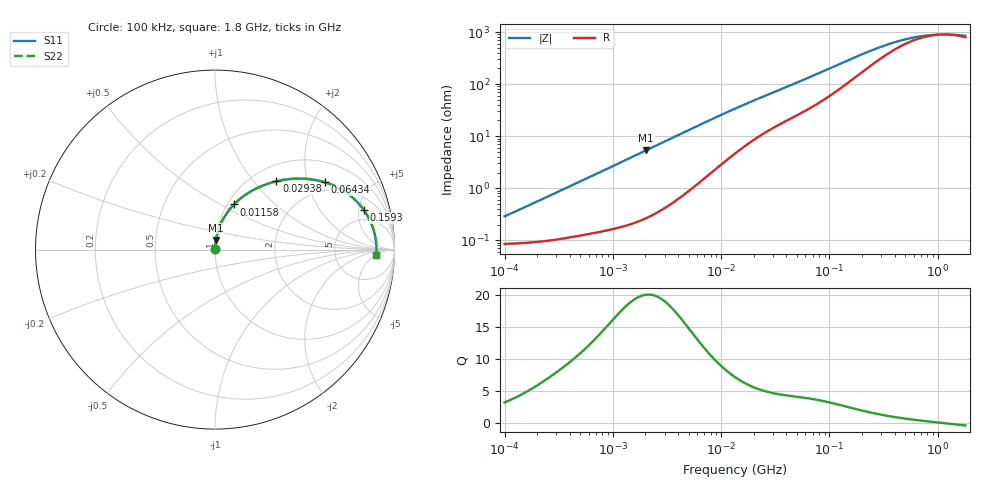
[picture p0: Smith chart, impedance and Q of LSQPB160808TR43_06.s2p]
! LSQPB160808TR43_06  S-PARAMETER MODEL  ( General Type )
! Model Generated by TAIYO YUDEN Corporation (http://www.ty-top.com)
! Version 1.0
! TAIYO YUDEN Control No. 110726NG25SE-FKC
! Copyright(c) 2011 TAIYO YUDEN CO.,LTD. All Rights Reserved.
! Product Description (link to TY-COMPAS)
! https://ds.yuden.co.jp/TYCOMPAS/or/detail?pn=LSQPB160808TR43M06&u=M
! Products Name : Inductors
! Characteristics :
!  Inductance : 0.43 uH , SRF(min) : 740 MHz , DC Resistance(max) : 0.1066 Ohm
!  Rated Current : Saturation :1400 mA , Temp Rise : 1100 mA (40 degC)
!  Case Size : 1.6 x 0.8 / 0.063 x 0.031 [mm/inch] , Thickness : 0.8 / 0.031 [mm/inch]
!  (Conditions: Temperature = 25 degC , DC Bias Current/Voltage = 0A / 0V)
! External Node Assignments :
!  1  o---GGG---o  2
! GND o---------o GND
! Frequency Range : 0.1MHz  -  1800MHz  [ 402 STEP ]
# MHz S RI R 50
! Freq[MHz].  S11 Real  S11 Imag  S21 Real  S21 Imag  S12 Real  S12 Imag  S22 Real  S22 Imag
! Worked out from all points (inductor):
!   401 points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, 100 kHz to 1.8 GHz, reference 50 ohm
!   read as one part in series: L = 438 nH near 105 kHz
!   highest Q = 20.1 at 2.035 MHz (marker M1), where L = 419 nH
!   self-resonance near 1.146 GHz
!   S11 on the Smith chart (normalised r, x): 100 kHz: 1.00, +0.01; 11.58 MHz: 1.07, +0.58; 29.38 MHz: 1.28, +1.32; 64.34 MHz: 1.67, +2.59; 159.3 MHz: 3.37, +5.64; 1.8 GHz: 17, -6
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0.1  0.000857 0.00275  0.9991 -0.00275  0.9991 -0.00275  0.000857 0.00275
0.144402  0.000896 0.00397  0.9991 -0.00397  0.9991 -0.00397  0.000896 0.00397
0.516129  0.00144 0.0139  0.9986 -0.0139  0.9986 -0.0139  0.00144 0.0139
2.034681  0.0055 0.0531  0.9945 -0.0531  0.9945 -0.0531  0.0055 0.0531
2.66389  0.00837 0.0692  0.9916 -0.0692  0.9916 -0.0692  0.00837 0.0692
6.278453  0.0375 0.1548  0.9625 -0.1548  0.9625 -0.1548  0.0375 0.1548
8.632747  0.0655 0.2024  0.9345 -0.2024  0.9345 -0.2024  0.0655 0.2024
11.58263  0.106 0.2517  0.894 -0.2517  0.894 -0.2517  0.106 0.2517
13.41641  0.1327 0.2769  0.8673 -0.2769  0.8673 -0.2769  0.1327 0.2769
19.37354  0.2183 0.3346  0.7817 -0.3346  0.7817 -0.3346  0.2183 0.3346
29.38042  0.3426 0.3806  0.6574 -0.3806  0.6574 -0.3806  0.3426 0.3806
44.5561  0.4853 0.3956  0.5147 -0.3956  0.5147 -0.3956  0.4853 0.3956
64.33982  0.6134 0.3747  0.3866 -0.3747  0.3866 -0.3747  0.6134 0.3747
69.24595  0.6375 0.3665  0.3625 -0.3665  0.3625 -0.3665  0.6375 0.3665
105.0131  0.754 0.3005  0.246 -0.3005  0.246 -0.3005  0.754 0.3005
159.2548  0.8284 0.2216  0.1716 -0.2216  0.1716 -0.2216  0.8284 0.2216
229.9669  0.8648 0.1588  0.1352 -0.1588  0.1352 -0.1588  0.8648 0.1588
357.3983  0.8863 0.0992  0.1137 -0.0992  0.1137 -0.0992  0.8863 0.0992
542.0029  0.8953 0.057  0.1047 -0.057  0.1047 -0.057  0.8953 0.057
802.0705  0.8988 0.0254  0.1012 -0.0254  0.1012 -0.0254  0.8988 0.0254
1186.925  0.8998 -0.00247  0.1002 0.00247  0.1002 0.00247  0.8998 -0.00247
1800  0.8987 -0.0326  0.1013 0.0326  0.1013 0.0326  0.8987 -0.0326
